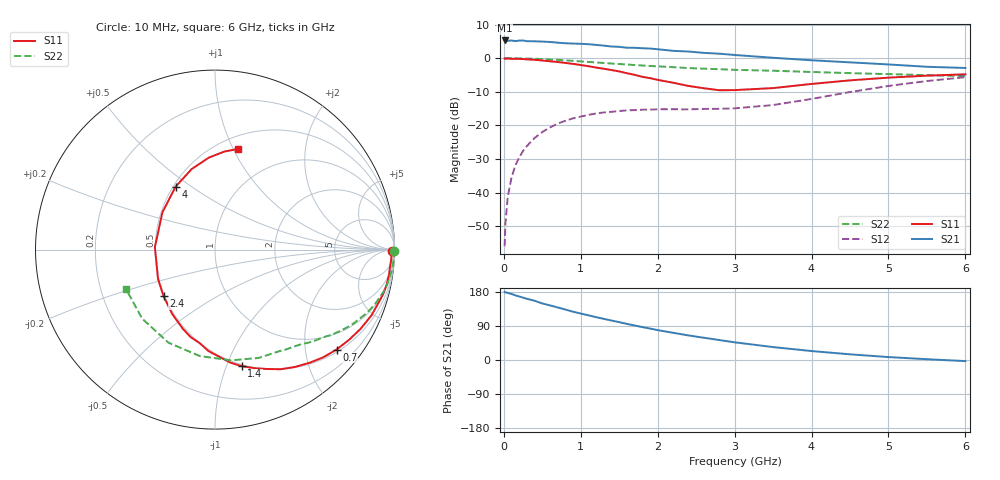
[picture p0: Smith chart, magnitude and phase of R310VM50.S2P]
! SIEMENS Small Signal Semiconductors
! BFR181
! Si NPN RF Bipolar Junction Transistor in SOT23
! VCE = 10 V  IC = 0.5 mA
! Common Emitter S-Parameters:  May  1996
# GHz  S  MA  R  50
!  f  S11  S21  S12  S22
! GHz  MAG  ANG  MAG  ANG  MAG  ANG  MAG  ANG
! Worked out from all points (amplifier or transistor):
!   36 points, 10 MHz to 6 GHz, reference 50 ohm
!   highest |S21| = 5.3 dB at 10 MHz (marker M1)
!   |S21| within 3 dB of that: start of sweep to 2.163 GHz
!   unconditionally stable (mu >= 1): 2.423 GHz to 4.004 GHz
!   at 250 MHz: K = 0.11, MSG = 16.4 dB, |S12| = -27.6 dB
!   at 1.4 GHz: K = 0.59, MSG = 9.7 dB, |S12| = -16.0 dB
!   at 6 GHz: K = 0.91, MSG = 1.4 dB, |S12| = -5.7 dB
!   S11 on the Smith chart (normalised r, x): 10 MHz: open; 700 MHz: 0.56, -2.69; 1.4 GHz: 0.49, -1.13; 2.4 GHz: 0.49, -0.30; 4 GHz: 0.51, +0.44; 6 GHz: 0.62, +1.05
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0.01  0.9856 -0.5  1.835 179.7  0.0016 91.9  0.999 -0.3
0.02  0.9823 -1.2  1.794 178.6  0.0034 87.7  0.994 -0.6
0.05  0.9841 -2.9  1.813 177.1  0.0085 88.7  0.9988 -1.4
0.1  0.9798 -5.6  1.833 174.4  0.0169 87.2  0.9989 -2.7
0.15  0.9795 -8.3  1.794 170.5  0.0254 82.8  0.9954 -4.2
0.25  0.9697 -14.6  1.832 164.6  0.0418 79.8  0.9915 -7.0
0.4  0.946 -22.7  1.784 156.3  0.065 74.0  0.9798 -11.0
0.5  0.9234 -28.6  1.766 149.2  0.0798 70.2  0.9694 -13.7
0.7  0.8769 -39.4  1.701 138.7  0.1061 63.0  0.9433 -18.5
0.9  0.8224 -50.0  1.65 127.4  0.1275 56.3  0.9133 -23.1
1.1  0.76 -61.3  1.614 117.9  0.1437 50.7  0.8803 -27.3
1.4  0.6662 -77.1  1.491 104.1  0.1594 43.6  0.8329 -33.0
1.9  0.5049 -105.8  1.391 83.0  0.1718 36.7  0.7655 -40.5
2.2  0.4314 -123.4  1.286 71.8  0.1739 35.0  0.7354 -44.8
2.4  0.3865 -137.8  1.256 64.8  0.1733 35.5  0.7131 -47.7
3  0.3352 177.7  1.116 46.7  0.1794 40.1  0.6711 -57.3
3.5  0.359 144.7  1.014 34.1  0.2009 46.4  0.6509 -68.0
4  0.4138 122.0  0.931 23.6  0.2477 51.0  0.6234 -81.8
4.5  0.4679 106.0  0.867 15.0  0.3137 50.2  0.5992 -98.1
5  0.5138 93.8  0.807 7.7  0.3863 45.7  0.5798 -116.6
5.5  0.5497 84.3  0.745 2.1  0.4574 38.4  0.5591 -136.5
6  0.5759 76.9  0.715 -2.9  0.5216 29.9  0.5425 -156.4
